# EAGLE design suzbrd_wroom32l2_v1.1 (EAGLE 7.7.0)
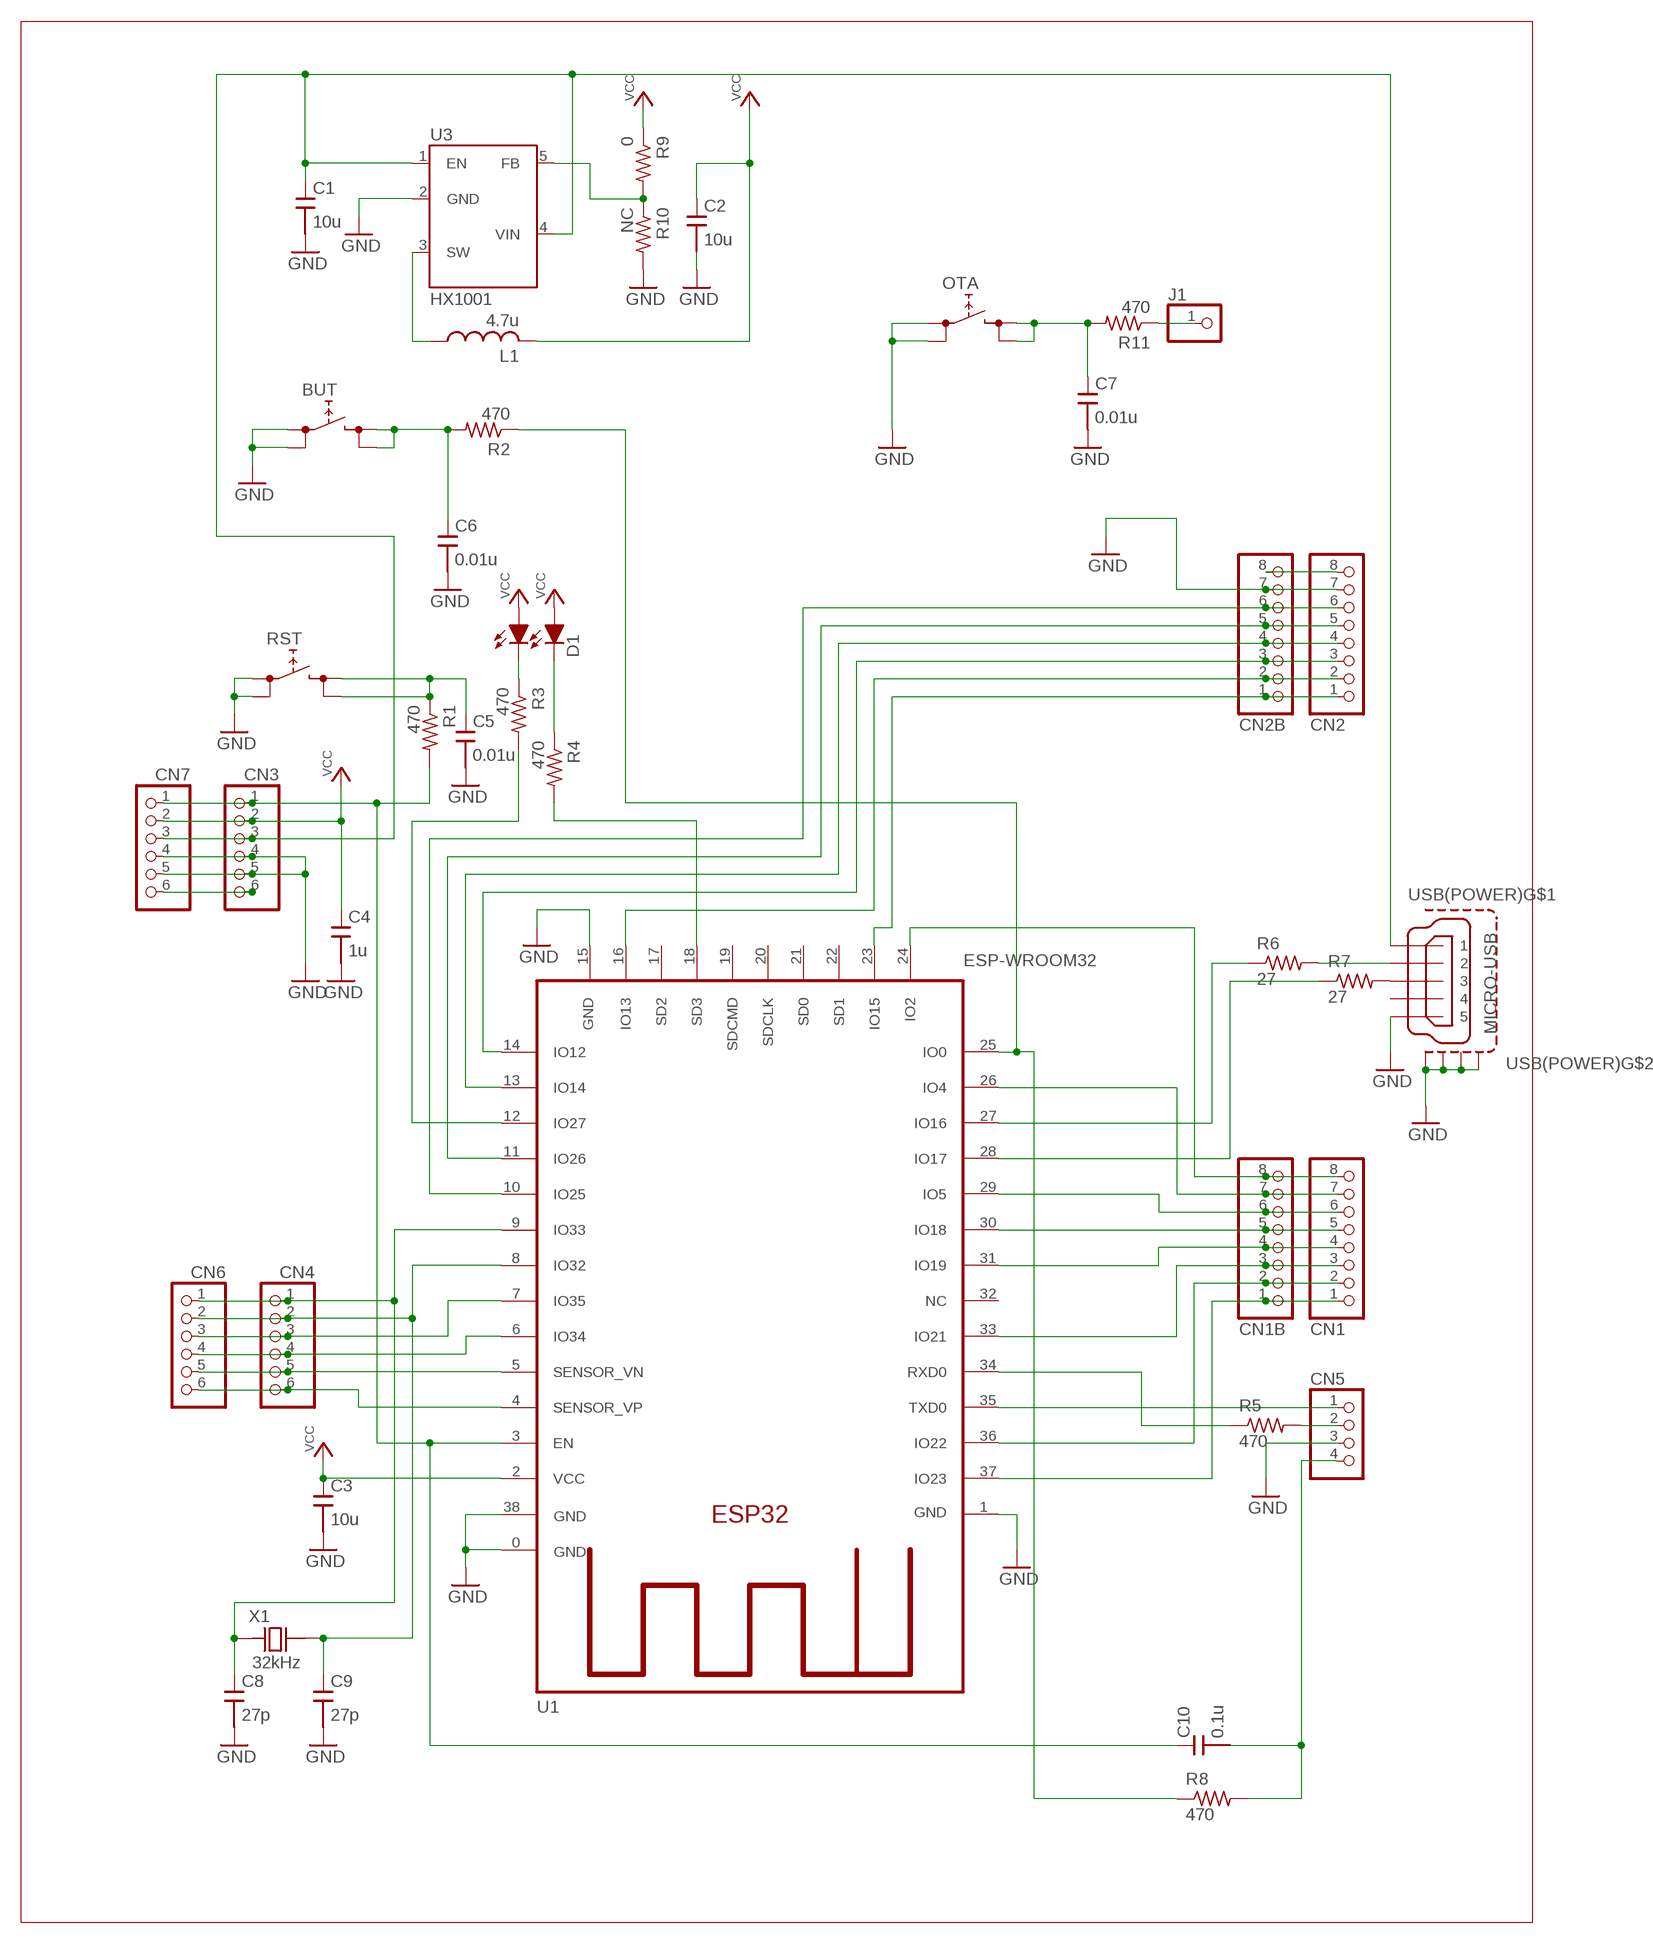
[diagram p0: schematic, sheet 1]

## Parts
BUT  TACTSWSMD+  [TACTSW/SMD+]
C1  10u  C/SMDC2012  [C2012]
C2  10u  C/SMDC2012  [C2012]
C3  10u  C/SMDC2012  [C2012]
C4  1u  C/SMDC2012  [C2012]
C5  0.01u  C/SMDC2012  [C2012]
C6  0.01u  C/SMDC2012  [C2012]
C7  0.01u  C/SMDC2012  [C2012]
C8  27p  C/SMDC2012  [C2012]
C9  27p  C/SMDC2012  [C2012]
C10  0.1u  C/SMDC2012  [C2012]
CN1  PINHDR8  [PINHDR1X8]
CN1B  PINHDR81.0  [PINHDR1X8_1.0]
CN2  PINHDR8  [PINHDR1X8]
CN2B  PINHDR81.0  [PINHDR1X8_1.0]
CN3  PINHDR61.0  [PINHDR1X6_1.0]
CN4  PINHDR61.0  [PINHDR1X6_1.0]
CN5  CONN4N  [PINHDR1X4]
CN6  PINHDR61.0  [PINHDR1X6_1.0]
CN7  PINHDR61.0  [PINHDR1X6_1.0]
D1  SEC2XX4  [LED3025]
J1  PINHDR1S  [PINHDRS1]
L1  4.7u  L/SMDCD43  [CD43]
OTA  TACTSWSMD+  [TACTSW/SMD+]
R1  470  R/SMDR2012  [R2012]
R2  470  R/SMDR2012  [R2012]
R3  470  R/SMDR2012  [R2012]
R4  470  R/SMDR2012  [R2012]
R5  470  R/SMDR2012  [R2012]
R6  27  R/SMDR2012  [R2012]
R7  27  R/SMDR2012  [R2012]
R8  470  R/SMDR2012  [R2012]
R9  0  R/SMDR2012  [R2012]
R10  NC  R/SMDR2012  [R2012]
R11  470  R/SMDR2012  [R2012]
RST  TACTSWSMD+  [TACTSW/SMD+]
U1  ESP-WROOM32  [ESP-WROOM32]
U3  HX1001  [SOT235]
USB(POWER)  MICRO-USB  [ZX62R]
X1  32kHz  CRYSTALFC255  [FC255]

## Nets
5V: C1.1 CN3.3 CN7.3 U3.1(EN) U3.4(VIN) USB(POWER).1
EN: C10.1 CN3.1 CN7.1 R1.2 U1.3(EN)
GND: BUT.1 BUT.2 C1.2 C2.2 C3.2 C4.2 C5.2 C6.2 C7.2 C8.2 C9.2 CN2.7 CN2B.7 CN3.4 CN3.5 CN5.3 CN7.4 CN7.5 OTA.1 OTA.2 R10.2 RST.1 RST.2 U1.0(GND) U1.1(GND) U1.15(GND) U1.38(GND) U3.2(GND) USB(POWER).5 USB(POWER).M1(S1) USB(POWER).M2(S2) USB(POWER).M3(S3) USB(POWER).M4(S4)
IO0: R2.1 R8.1 U1.25(IO0)
IO2: CN1.8 CN1B.8 U1.24(IO2)
IO4: CN1.7 CN1B.7 U1.26(IO4)
IO5: CN1.6 CN1B.6 U1.29(IO5)
IO12: CN2.3 CN2B.3 U1.14(IO12)
IO13: CN2.2 CN2B.2 U1.16(IO13)
IO14: CN2.4 CN2B.4 U1.13(IO14)
IO15: CN2.1 CN2B.1 U1.23(IO15)
IO16: R6.1 U1.27(IO16)
IO17: R7.1 U1.28(IO17)
IO18: CN1.5 CN1B.5 U1.30(IO18)
IO19: CN1.4 CN1B.4 U1.31(IO19)
IO21: CN1.3 CN1B.3 U1.33(IO21)
IO22: CN1.2 CN1B.2 U1.36(IO22)
IO23: CN1.1 CN1B.1 U1.37(IO23)
IO25: CN2.6 CN2B.6 U1.10(IO25)
IO26: CN2.5 CN2B.5 U1.11(IO26)
IO27: R3.2 U1.12(IO27)
IO32: C9.1 CN4.2 CN6.2 U1.8(IO32) X1.2
IO33: C8.1 CN4.1 CN6.1 U1.9(IO33) X1.1
IO34: CN4.4 CN6.4 U1.6(IO34)
IO35: CN4.3 CN6.3 U1.7(IO35)
N$1: R7.2 USB(POWER).3
N$3: CN5.2 R5.2
N$4: C10.2 CN5.4 R8.2
N$5: R9.2 R10.1 U3.5(FB)
N$6: CN3.6 CN7.6
N$7: C7.1 OTA.3 OTA.4 R11.2
N$8: J1.1 R11.1
N$21: C5.1 R1.1 RST.3 RST.4
N$25: D1.2(C1) R3.1
N$26: D1.1(C0) R4.1
N$28: R4.2 U1.18(SD3)
N$32: R6.2 USB(POWER).2
N$36: CN2.8 CN2B.8
N$37: BUT.3 BUT.4 C6.1 R2.2
RXD0: R5.1 U1.34(RXD0)
SW: L1.1 U3.3(SW)
TXD0: CN5.1 U1.35(TXD0)
VCC: C2.1 C3.1 C4.1 CN3.2 CN7.2 D1.3(A1) D1.4(A0) L1.2 R9.1 U1.2(VCC)
VN: CN4.5 CN6.5 U1.5(SENSOR_VN)
VP: CN4.6 CN6.6 U1.4(SENSOR_VP)
Unconnected: U1.17(SD2) U1.19(SDCMD) U1.20(SDCLK) U1.21(SD0) U1.22(SD1) U1.32(NC) USB(POWER).4

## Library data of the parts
BUT OTA RST = SRT162-010:TACTSW: 4pin tactsw (1,2 - 3,4)
C1-C10 = SRT162-010:C/SMD
CN1 CN1B CN2 CN2B = SRT162-010:PINHDR8
CN3 CN4 CN6 CN7 = SRT162-010:PINHDR6
CN5 = SRT162-010:CONN4: connector 4
D1 = SRT162-010:SEC2XX4
J1 = SRT162-020:PINHDR1
L1 = SRT162-020:L/SMD: VLF4012AT
R1-R11 = SRT162-010:R/SMD
U1 = SRT162-020:ESP-WROOM32
U3 = SRT162-010:HX1001
USB(POWER) = SRT162-020:MICRO-USB
X1 = SRT162-020:CRYSTAL

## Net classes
1 Power: width 0.381 mm, clearance 0.203 mm to class 0

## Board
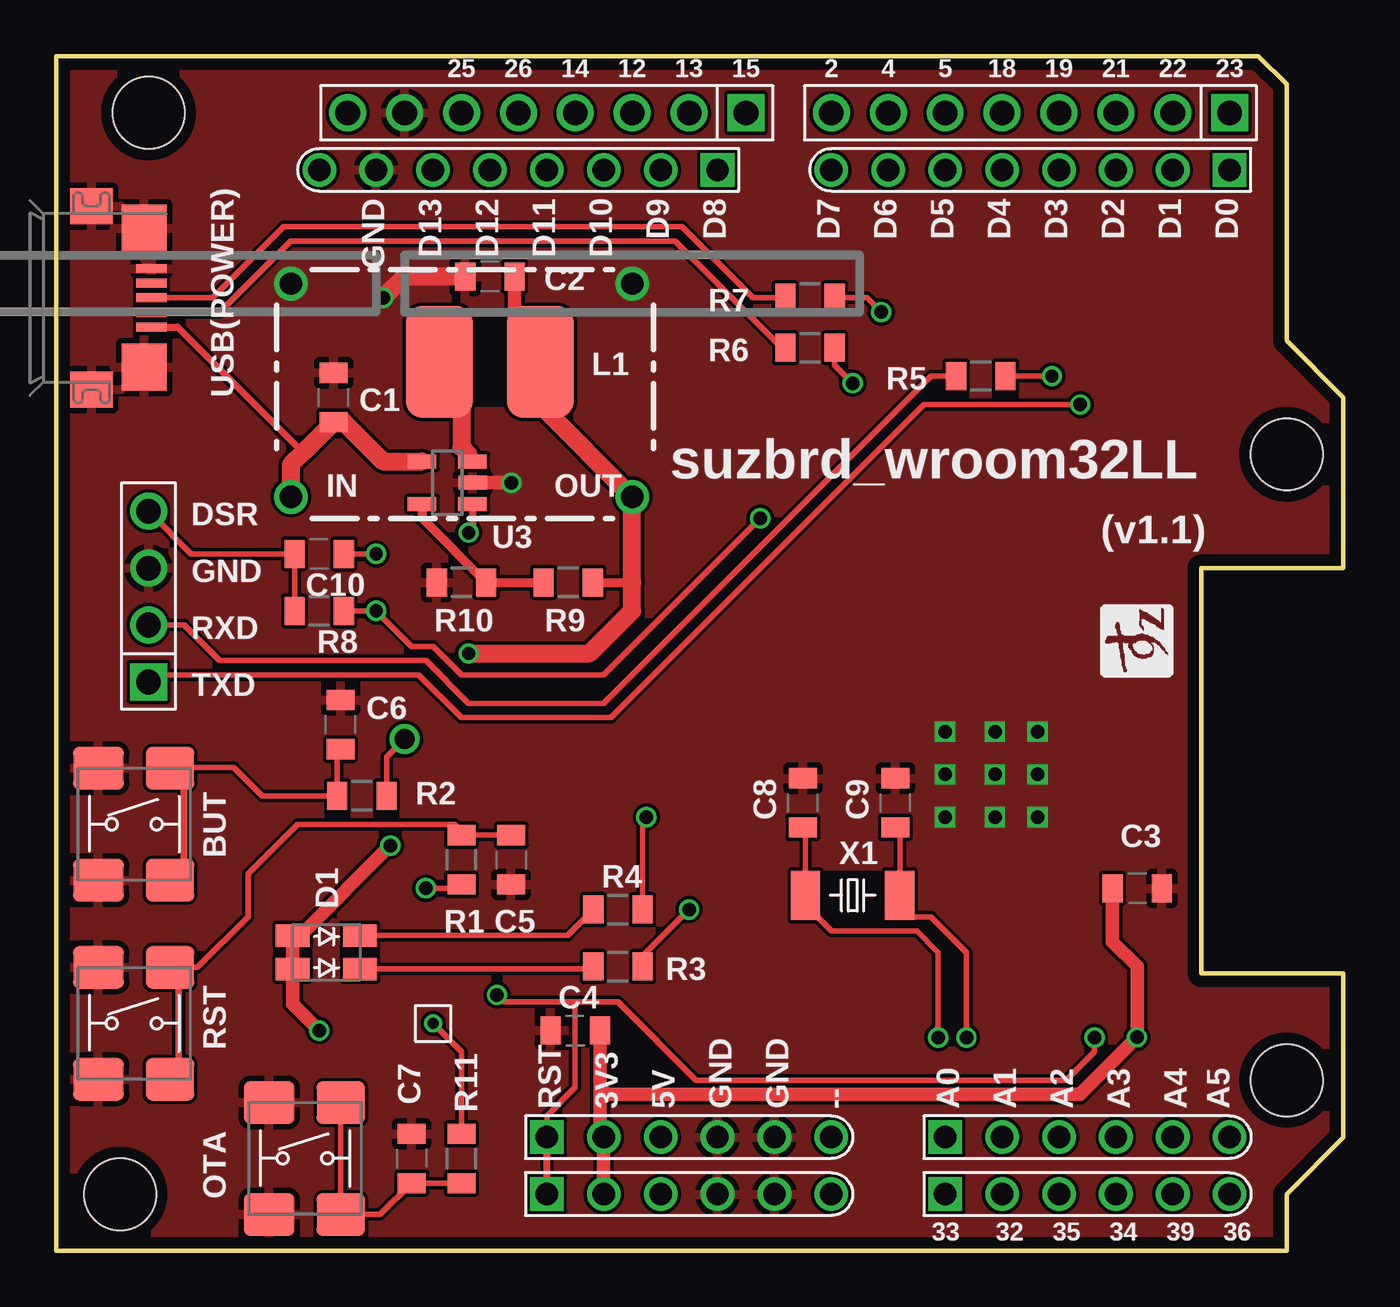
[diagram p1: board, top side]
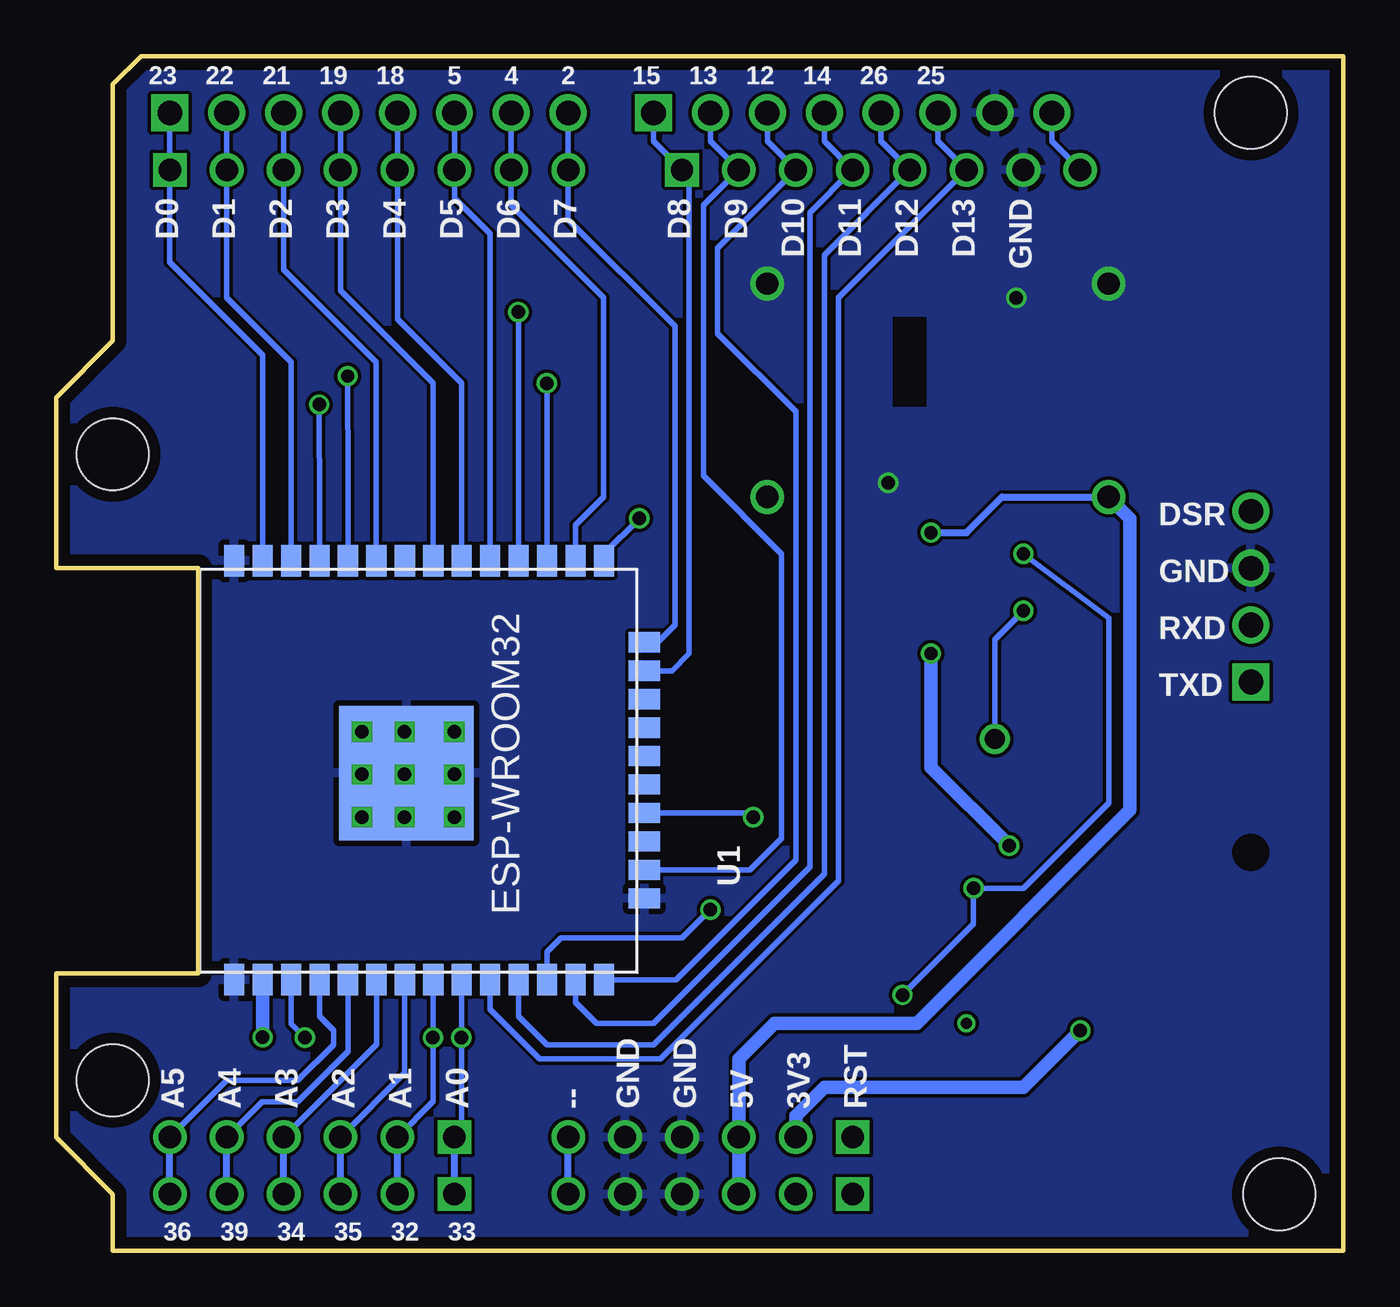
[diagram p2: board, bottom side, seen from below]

Size 57.47 x 53.34 mm. Coordinates in mm from the lower left corner, seen from the top.
Outline: 0,0 54.93,0 54.93,2.54 57.47,5.08 57.47,12.38 51.12,12.38 51.12,30.48 57.47,30.48 57.47,38.1 54.93,40.64 54.93,52.07 53.66,53.34 0,53.34 0,0
Copper layers (1*16): Top 0.035mm / dielectric 1.6mm / Bottom 0.035mm
Design rules "Elecrow_2-layer_PCB_eagle_rule": minimum track width 6mil, minimum drill 12mil, track to track 6mil, track to pad 6mil, pad to pad 6mil, via to via 8mil, smd to smd 0mil, copper to edge 20mil, drill to drill 10mil, minimum pad ring 6mil, minimum via ring 6mil, stop-mask expansion 0mil, vias tented up to drill 100mil, thermal gap 10mil
Holes 3.2 mm at 54.93,7.62 54.93,35.56 2.86,2.54 4.13,50.8
bRestrict: area 3.8,17.5 to 4.4,18.1
vRestrict: area -7.9,37.5 to 35.9,40; area 2.9,-1.3 to 34.6,0.6

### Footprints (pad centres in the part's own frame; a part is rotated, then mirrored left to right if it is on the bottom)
TACTSW/SMD+ = smd 2.25 x 1.9: 1 -1.6,2.5; 2 -1.6,-2.5 | smd 2.15 x 1.9: 3 1.6,2.5; 4 1.6,-2.5
C2012 = smd 0.9 x 1.25: 1 -1.1,0; 2 1.1,0
PINHDR1X8 = drill 1.1 square: 1 -8.89,0 | drill 1.1: 2 -6.35,0; 3 -3.81,0; 4 -1.27,0; 5 1.27,0; 6 3.81,0; 7 6.35,0; 8 8.89,0
PINHDR1X8_1.0 = drill 1 square: 1 -8.89,0 | drill 1: 2 -6.35,0; 3 -3.81,0; 4 -1.27,0; 5 1.27,0; 6 3.81,0; 7 6.35,0; 8 8.89,0
PINHDR1X6_1.0 = drill 1 square: 1 -6.35,0 | drill 1: 2 -3.81,0; 3 -1.27,0; 4 1.27,0; 5 3.81,0; 6 6.35,0
PINHDR1X4 = drill 1.1 square: 1 -3.81,0 | drill 1.1: 2 -1.27,0; 3 1.27,0; 4 3.81,0
LED3025 = smd 1.5 x 1: 1 1.5,0.75; 2 1.5,-0.75; 3 -1.5,-0.75; 4 -1.5,0.75
PINHDRS1 = drill 0.5: 1 0,0
CD43 = smd 3 x 5: 1 -2.25,0; 2 2.25,0
R2012 = smd 0.9 x 1.25: 1 -1.1,0; 2 1.1,0
ESP-WROOM32 = smd 6 x 6: 0 9.9,12.3 | smd 1.4 x 0.9: 1 0.68,19.99; 2 0.68,18.72; 3 0.68,17.45; 4 0.68,16.18; 5 0.68,14.91; 6 0.68,13.64; 7 0.68,12.37; 8 0.68,11.1; 9 0.68,9.83; 10 0.68,8.56; 11 0.68,7.29; 12 0.68,6.02; 13 0.68,4.75; 14 0.68,3.48; 25 19.38,3.48; 26 19.38,4.75; 27 19.38,6.02; 28 19.38,7.29; 29 19.38,8.56; 30 19.38,9.83; 31 19.38,11.1; 32 19.38,12.37; 33 19.38,13.64; 34 19.38,14.91; 35 19.38,16.18; 36 19.38,17.45; 37 19.38,18.72; 38 19.38,19.99 | smd 0.9 x 1.4: 15 4.31,1.68; 16 5.58,1.68; 17 6.85,1.68; 18 8.12,1.68; 19 9.39,1.68; 20 10.66,1.68; 21 11.93,1.68; 22 13.2,1.68; 23 14.47,1.68; 24 15.74,1.68
SOT235 = smd 0.635 x 1.27: 1 -0.95,-1.125; 2 0.013,-1.135; 3 0.95,-1.125; 4 0.95,1.125; 5 -0.95,1.125
ZX62R = smd 1.35 x 0.4: 1 2.675,-1.3; 2 2.675,-0.65; 3 2.675,0; 4 2.675,0.65; 5 2.675,1.3 | smd 1.9 x 1.6: M1 0,-4.1; M2 0,4.1 | smd 2 x 2.1: M3 2.35,3.1; M4 2.35,-3.1
FC255 = smd 1.3 x 2.2: 1 2.1,0; 2 -2.1,0

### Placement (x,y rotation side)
BUT  3.49,19.05 0 top
C1  12.38,38.1 90 top
C2  19.37,43.5 180 top
C3  48.26,16.19 0 top
C4  23.18,9.84 180 top
C5  20.32,17.46 270 top
C6  12.7,23.49 90 top
C7  15.88,4.13 90 top
C8  33.34,20 90 top
C9  37.47,20 90 top
C10  11.75,31.11 180 top
CN1  43.5,50.8 180 top
CN1B  43.5,48.26 180 top
CN2  21.91,50.8 180 top
CN2B  20.64,48.26 180 top
CN3  28.26,5.08 0 top
CN4  46.04,5.08 0 top
CN5  4.13,29.21 90 top
CN6  46.04,2.54 0 top
CN7  28.26,2.54 0 top
D1  12.06,13.33 0 top
J1  16.83,10.16 0 top
L1  19.37,39.69 0 top
OTA  11.11,4.13 0 top
R1  18.1,17.46 270 top
R2  13.65,20.32 180 top
R3  25.08,12.7 0 top
R4  25.08,15.24 0 top
R5  41.28,39.05 180 top
R6  33.66,40.32 180 top
R7  33.66,42.55 180 top
R8  11.75,28.57 180 top
R9  22.86,29.85 180 top
R10  18.1,29.85 180 top
R11  18.1,4.13 270 top
RST  3.49,10.16 0 top
U1  29.53,11.43 90 bottom
U3  17.46,34.29 90 top
USB(POWER)  1.59,42.55 0 top
X1  35.56,15.88 180 top

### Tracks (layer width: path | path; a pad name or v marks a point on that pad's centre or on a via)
5V  (via drill 0.6, 1)
  Top 0.305: U3.1 18.59,32.24 v18.41,32.07 | USB(POWER).1 5.43,41.25 11.03,35.65
  Top 0.406: 10.48,34.61 v10.48,33.66
  Top 0.813: U3.4 14.61,35.24 12.85,37 C1.1 11.03,35.65 10.48,35.1 v10.48,33.66
  Bottom 0.305: v18.41,32.07 16.83,32.07 15.24,33.66 v10.48,33.66
  Bottom 0.61: v10.48,33.66 9.52,32.7 9.52,19.68 19.05,10.16 25.4,10.16 26.99,8.57 CN3.3 CN7.3
EN  (via drill 0.6)
  Top 0.254: R1.2 17.93,16.19 v16.51,16.19 | C10.1 v14.29,31.11 | CN3.1 21.91,6.03 23.18,7.3 23.18,11.11 | v46.36,9.52 46.36,8.89 45.08,7.62 28.58,7.62 25.08,11.11 23.18,11.11 | 23.18,11.11 20,11.11 v19.68,11.43
  Top 0.305: CN7.1 CN3.1
  Bottom 0.254: v14.29,31.11 10.48,28.26 10.48,20 14.29,16.19 v16.51,16.19 16.51,14.61 v19.68,11.43 | U1.3 46.98,10.15 v46.36,9.52
  Bottom 0.3: CN3.1
GND  (via drill 0.6, 1)
  Top 0.406: 49.53,16.02 C3.2
  Top 0.61: U3.2 20.31,34.3 v20.32,34.29
  Top 0.813: C2.2 15.56,43.5 v14.61,42.55
  other vias: 43.81,19.37 43.81,23.18 39.69,23.18 39.69,19.37 41.91,21.27 41.91,19.37 39.69,21.27 43.81,21.27 41.91,23.18 10.48,43.18 25.72,43.18
  pour Bottom: -10.48,54.61 60.01,54.61 60.01,-2.54 -10.48,-2.54
  pour Top: -11.11,55.88 61.28,55.88 61.28,-3.17 -11.11,-3.17
IO0  (via drill 0.6, 0.9)
  Top 0.254: R8.1 v14.29,28.57 15.88,26.99 16.83,26.99 18.1,25.72 24.45,25.72 v31.43,32.7 | R2.1 14.75,22.05 v15.56,22.86
  Bottom 0.254: U1.25 33.01,31.13 v31.43,32.7 | v14.29,28.57 15.56,27.3 v15.56,22.86
IO2
  Bottom 0.254: U1.24 30.61,27.17 29.85,27.94 29.85,41.28 34.61,46.04 CN1B.8 CN1.8
IO4
  Bottom 0.254: U1.26 34.28,32.4 33.02,33.66 33.02,42.55 37.15,46.67 CN1B.7 CN1.7
IO5
  Bottom 0.254: U1.29 38.1,30.82 38.1,45.4 39.69,46.99 CN1B.6 | 39.69,47.94 CN1B.6 | CN1B.6 CN1.6
IO12
  Bottom 0.254: U1.14 29.8,12.11 24.45,17.46 24.45,37.47 27.94,40.96 27.94,44.77 CN2B.3 25.72,49.53 CN2.3
IO13
  Bottom 0.254: CN2.2 28.26,49.53 CN2B.2 28.58,46.67 28.58,34.61 25.08,31.11 25.08,18.41 26.49,17.01 U1.16
IO14
  Bottom 0.254: U1.13 34.28,11.1 33.34,10.16 30.8,10.16 23.81,17.14 23.81,46.36 CN2B.4 23.18,49.53 CN2.4
IO15
  Bottom 0.254: U1.23 29.98,25.9 29.21,26.67 29.21,47.94 CN2B.1 30.8,49.53 CN2.1
IO16  (via drill 0.6)
  Top 0.254: R6.1 34.75,39.54 v35.56,38.73
  Bottom 0.254: U1.27 35.55,33.67 v35.56,38.73
IO17  (via drill 0.6)
  Top 0.254: R7.1 36.19,42.55 v36.83,41.91
  Bottom 0.254: 36.83,30.82 U1.28 36.82,41.9 v36.83,41.91
IO18
  Bottom 0.254: U1.30 39.37,30.82 39.37,38.73 42.23,41.59 CN1B.5 CN1.5
IO19
  Bottom 0.254: U1.31 40.64,30.82 40.64,38.73 44.77,42.86 CN1B.4 CN1.4
IO21
  Bottom 0.254: U1.33 43.18,30.82 43.18,39.69 47.31,43.82 CN1B.3 CN1.3
IO22
  Bottom 0.254: CN1.2 CN1B.2 49.85,42.55 46.98,39.68 U1.36
IO23
  Bottom 0.254: CN1.1 CN1B.1 52.39,44.13 48.25,39.99 U1.37
IO25
  Bottom 0.254: U1.10 38.09,10.78 35.88,8.57 30.48,8.57 22.54,16.51 22.54,42.55 CN2B.6 18.1,49.53 CN2.6
IO26
  Bottom 0.254: U1.11 36.82,10.46 35.56,9.21 30.8,9.21 23.18,16.83 23.18,44.45 CN2B.5 20.64,49.53 CN2.5
IO27  (via drill 0.6)
  Top 0.254: R3.2 26.18,13.16 v28.26,15.24
  Bottom 0.254: U1.12 35.55,13.35 34.93,13.97 29.53,13.97 v28.26,15.24
IO32  (via drill 0.6)
  Top 0.254: C9.1 37.66,18.71 X1.2 37.66,15.36 38.1,14.92 39.05,14.92 40.64,13.33 v40.64,9.52
  Bottom 0.254: CN4.2 40.63,6.68 U1.8 40.63,9.54 v40.64,9.52
  Bottom 0.305: CN6.2 CN4.2
IO33  (via drill 0.6)
  Top 0.254: C8.1 33.46,18.78 X1.1 33.46,15.43 34.61,14.29 38.42,14.29 39.37,13.33 v39.37,9.52
  Bottom 0.254: CN4.1 39.36,5.41 U1.9 39.36,9.54 v39.37,9.52
  Bottom 0.305: CN6.1 CN4.1
IO34
  Bottom 0.254: U1.6 43.17,9.22 CN4.4
  Bottom 0.305: CN6.4 CN4.4
IO35
  Bottom 0.254: U1.7 41.9,7.95 CN4.3
  Bottom 0.305: CN6.3 CN4.3
N$1
  Top 0.254: USB(POWER).3 6.99,42.55 10.16,45.72 27.94,45.72 31.11,42.55 R7.2
N$3
  Top 0.254: CN5.2 5.72,27.94 7.3,26.35 16.51,26.35 18.41,24.45 24.45,24.45 39.05,39.05 R5.2
N$4
  Top 0.254: R8.2 C10.2 6.03,31.11 CN5.4
N$5
  Top 0.406: R9.2 R10.1 16.34,32.71 U3.5
N$6
  Bottom 0.305: CN7.6 CN3.6
N$7
  Top 0.254: R11.2 C7.1 14.47,1.63 OTA.4 OTA.3
N$8
  Top 0.254: R11.1 18.1,8.89 J1.1
N$21
  Top 0.254: 5.48,11.99 5.48,12.14 | C5.1 R1.1 18.25,18.41 18.41,18.41 17.78,19.05 10.79,19.05 8.57,16.83 8.57,14.92 6.31,12.66 RST.3
  Top 0.3: RST.4 5.48,7.86 5.48,11.99 RST.3
N$25
  Top 0.254: D1.2 23.87,12.58 R3.1
N$26
  Top 0.254: D1.1 22.83,14.08 R4.1
N$28  (via drill 0.6)
  Top 0.254: R4.2 26.18,19.2 v26.35,19.37
  Bottom 0.254: U1.18 26.54,19.55 v26.35,19.37
N$32
  Top 0.254: USB(POWER).2 7.29,41.9 10.48,45.09 27.62,45.09 32.39,40.32 R6.2
N$36
  Bottom 0.254: CN2B.8 13.02,49.53 CN2.8
N$37
  Top 0.152: BUT.4 5.16,16.59 5.64,16.59 5.64,16.75 5.72,16.83
  Top 0.254: C6.1 12.55,22.25 R2.2 9.21,20.32 7.94,21.59 5.13,21.59 BUT.3
  Top 0.305: BUT.3 5.72,21.55 5.72,16.83
RXD0  (via drill 0.6)
  Top 0.254: v44.45,39.05 R5.1
  Bottom 0.254: U1.34 44.44,34.28 v44.45,39.05
SW
  Top 0.61: 18.41,35.56 18.41,35.41 U3.3
  Top 0.813: L1.1 18.1,38.71 18.1,35.88 18.41,35.56
TXD0  (via drill 0.6)
  Top 0.254: CN5.1 4.44,25.72 16.19,25.72 18.1,23.81 24.76,23.81 38.73,37.78 v45.72,37.78
  Bottom 0.254: U1.35 45.71,33.01 v45.72,37.78
VCC  (via drill 0.6, 1)
  Top 0.406: 20.47,39.67 L1.2 | R9.1 25.72,29.85
  Top 0.61: C2.1 20.47,39.67 | CN7.2 CN3.2 24.28,5.25 24.28,7.3 | C4.1 24.28,7.3 | 24.28,7.3 24.6,6.99 45.69,6.99 v48.25,9.54 48.26,9.55 48.26,12.7 47.16,13.8 C3.1 | v11.75,9.84 10.56,11.02 D1.3 D1.4 10.91,14.08 v14.92,18.1
  Top 0.813: L1.2 21.62,37.76 v25.72,33.66 25.72,29.85 25.72,28.57 23.81,26.67 v18.41,26.67
  Bottom 0.61: v14.92,18.1 18.41,21.59 v18.41,26.67 | U1.2 v48.25,9.54 | CN3.2 24.45,6.03 23.18,7.3 14.29,7.3 v11.75,9.84
VN
  Bottom 0.254: U1.5 44.44,8.9 46.67,6.67 48.26,6.67 CN4.5
  Bottom 0.305: CN6.5 CN4.5
VP
  Bottom 0.254: 52.06,5.41 CN4.6 49.85,7.62 46.67,7.62 45.08,9.21 45.08,9.84 45.71,10.46 U1.4
  Bottom 0.305: CN6.6 CN4.6

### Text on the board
tPlace: 25 | 26 | 14 | 12 | 13 | 15 | 2 | 4 | 5 | 18 | 19 | 21 | 22 | 23 | GND | D13 | D12 | D11 | D10 | D9 | D8 | D7 | D6 | D5 | D4 | D3 | D2 | D1 | D0 | suzbrd_wroom32LL | IN | OUT | DSR | (v1.1) | GND | RXD | TXD | RST | 3V3 | 5V | GND | GND | -- | A0 | A1 | A2 | A3 | A4 | A5 | 33 | 32 | 35 | 34 | 39 | 36
bPlace: 25 | 26 | 14 | 12 | 13 | 15 | 2 | 4 | 5 | 18 | 19 | 21 | 22 | 23 | GND | D13 | D12 | D11 | D10 | D9 | D8 | D7 | D6 | D5 | D4 | D3 | D2 | D1 | D0 | DSR | GND | RXD | TXD | RST | 3V3 | 5V | GND | GND | -- | A0 | A1 | A2 | A3 | A4 | A5 | 33 | 32 | 35 | 34 | 39 | 36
